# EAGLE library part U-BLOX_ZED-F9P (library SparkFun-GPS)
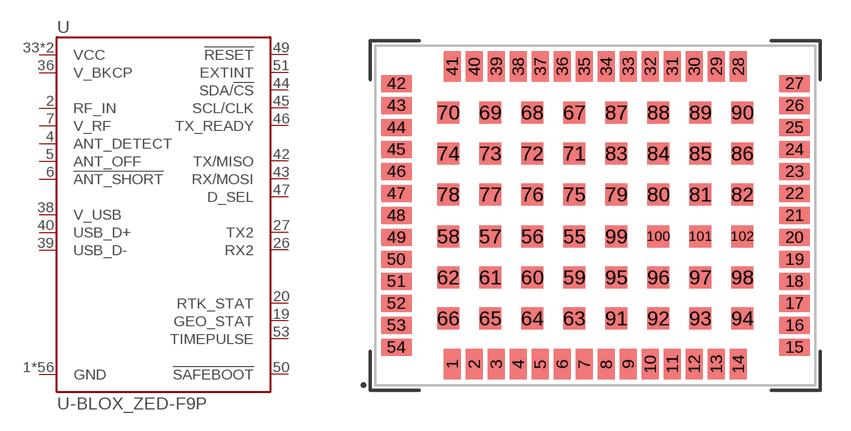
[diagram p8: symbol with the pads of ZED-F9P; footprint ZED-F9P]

Designator prefix U

## U-BLOX_ZED-F9P (PROD_ID: IC-14209)  [ZED-F9P]
1  GND
2  RF_IN
3  GND
4  ANT_DETECT
5  ANT_OFF
6  !ANT_SHORT!
7  V_RF
12  GND
14  GND
19  GEO_STAT
20  RTK_STAT
26  RX2
27  TX2
32  GND
33  VCC
34  VCC
36  V_BKCP
37  GND
38  V_USB
39  USB_D-
40  USB_D+
41  GND
42  TX/MISO
43  RX/MOSI
44  SDA/!CS!
45  SCL/CLK
46  TX_READY
47  D_SEL
48  GND
49  !RESET!
50  !SAFEBOOT!
51  EXTINT
53  TIMEPULSE
55  GND
56  GND
57  GND
58  GND
59  GND
60  GND
61  GND
62  GND
63  GND
64  GND
65  GND
66  GND
67  GND
68  GND
69  GND
70  GND
71  GND
72  GND
73  GND
74  GND
75  GND
76  GND
77  GND
78  GND
79  GND
80  GND
81  GND
82  GND
83  GND
84  GND
85  GND
86  GND
87  GND
88  GND
89  GND
90  GND
91  GND
92  GND
93  GND
94  GND
95  GND
96  GND
97  GND
98  GND
99  GND
100  GND
101  GND
102  GND

## Footprint ZED-F9P (pad centres in mm)
smd 0.85 x 1.52: 1 -7.15,-7.45; 2 -6.05,-7.45; 3 -4.95,-7.45; 4 -3.85,-7.45; 5 -2.75,-7.45; 6 -1.65,-7.45; 7 -0.55,-7.45; 8 0.55,-7.45; 9 1.65,-7.45; 10 2.75,-7.45; 11 3.85,-7.45; 12 4.95,-7.45; 13 6.05,-7.45; 14 7.15,-7.45; 28 7.15,7.45; 29 6.05,7.45; 30 4.95,7.45; 31 3.85,7.45; 32 2.75,7.45; 33 1.65,7.45; 34 0.55,7.45; 35 -0.55,7.45; 36 -1.65,7.45; 37 -2.75,7.45; 38 -3.85,7.45; 39 -4.95,7.45; 40 -6.05,7.45; 41 -7.15,7.45
smd 1.52 x 0.85: 15 9.95,-6.6; 16 9.95,-5.5; 17 9.95,-4.4; 18 9.95,-3.3; 19 9.95,-2.2; 20 9.95,-1.1; 21 9.95,0; 22 9.95,1.1; 23 9.95,2.2; 24 9.95,3.3; 25 9.95,4.4; 26 9.95,5.5; 27 9.95,6.6; 42 -9.95,6.6; 43 -9.95,5.5; 44 -9.95,4.4; 45 -9.95,3.3; 46 -9.95,2.2; 47 -9.95,1.1; 48 -9.95,0; 49 -9.95,-1.1; 50 -9.95,-2.2; 51 -9.95,-3.3; 52 -9.95,-4.4; 53 -9.95,-5.5; 54 -9.95,-6.6
smd 1.1 x 1.1: 55 -1.05,-1.05; 56 -3.15,-1.05; 57 -5.25,-1.05; 58 -7.35,-1.05; 59 -1.05,-3.1; 60 -3.15,-3.1; 61 -5.25,-3.1; 62 -7.35,-3.1; 63 -1.05,-5.15; 64 -3.15,-5.15; 65 -5.25,-5.15; 66 -7.35,-5.15; 67 -1.05,5.15; 68 -3.15,5.15; 69 -5.25,5.15; 70 -7.35,5.15; 71 -1.05,3.1; 72 -3.15,3.1; 73 -5.25,3.1; 74 -7.35,3.1; 75 -1.05,1.05; 76 -3.15,1.05; 77 -5.25,1.05; 78 -7.35,1.05; 79 1.05,1.05; 80 3.15,1.05; 81 5.25,1.05; 82 7.35,1.05; 83 1.05,3.1; 84 3.15,3.1; 85 5.25,3.1; 86 7.35,3.1; 87 1.05,5.15; 88 3.15,5.15; 89 5.25,5.15; 90 7.35,5.15; 91 1.05,-5.15; 92 3.15,-5.15; 93 5.25,-5.15; 94 7.35,-5.15; 95 1.05,-3.1; 96 3.15,-3.1; 97 5.25,-3.1; 98 7.35,-3.1; 99 1.05,-1.05; 100 3.15,-1.05; 101 5.25,-1.05; 102 7.35,-1.05

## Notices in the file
Licensing: Creative Commons ShareAlike 4.0 International - https://creativecommons.org/licenses/by-sa/4.0
